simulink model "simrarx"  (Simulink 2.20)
settings: Solver=ode45  StartTime=0.0  StopTime=300  FixedStep=1  MaxStep=1  RelTol=1e-3  AbsTol=1e-6

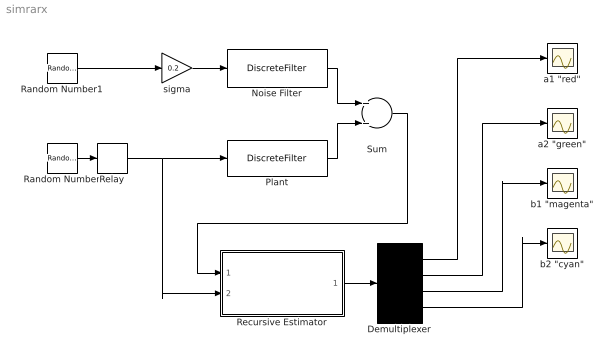
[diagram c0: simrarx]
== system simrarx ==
  Demultiplexer : Demux  Outputs=4
  Noise Filter : DiscreteFilter  Numerator=[1 -1 0.2]  Denominator=[1 -1.5 0.7]  SampleTime=1
  Plant : DiscreteFilter  Numerator=[1 0.5]  Denominator=[1 -1.5 0.7]  SampleTime=1
  Random Number : RandomNumber  Mean=0  Variance=1  Seed=123456789  SampleTime=1
  Random Number1 : RandomNumber  Mean=0  Variance=1  Seed=123459  SampleTime=1
  Recursive Estimator : Subsystem  mask(Recursive Estimator){nn=[2 2 1], ff=0.98, pdiag=10000, ts=1}
      mask prompts: nn "ARX model structure [na nb nk]  :"; ff "Forgetting factor  ff :"; pdiag "Íà÷àëíà ñòîéíîñò çà äèàãîíàëà íà êîâàðèàöèîííàòà ìàòðèöà  P  :"; ts "How often to sample points [sec] :"
      mask help: Recursive parameter estimation
      mask init:
      | nn=@1; ff=@2; pdiag=@3; ts=@4;
      | na=nn(1); d=na+nn(2); dm=sum(nn)-1;
      | i=[1:na  na+nn(3):dm];  ii=[1:dm];
  Relay : Relay  OnSwitchValue=eps  OffSwitchValue=eps  OnOutputValue=-1  OffOutputValue=1
  Sum : Sum  Inputs=++
  "a1 \"red\"" : Scope
  "a2 \"green\"" : Scope
  "b1 \"magenta\"" : Scope
  "b2 \"cyan\"" : Scope
  sigma : Gain  Gain=0.2
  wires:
  Random Number/1 -> Relay/1
  Random Number1/1 -> sigma/1
  sigma/1 -> Noise Filter/1
  Noise Filter/1 -> Sum/1
  Plant/1 -> Sum/2
  Sum/1 -> Recursive Estimator/1(y (k))
  Relay/1 -> Plant/1, Recursive Estimator/2(u (k))
  Recursive Estimator/1(tetha (k)) -> Demultiplexer/1
  Demultiplexer/1 -> "a1 \"red\""/1
  Demultiplexer/2 -> "a2 \"green\""/1
  Demultiplexer/3 -> "b1 \"magenta\""/1
  Demultiplexer/4 -> "b2 \"cyan\""/1

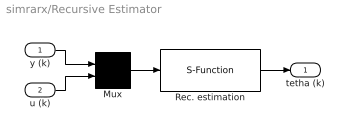
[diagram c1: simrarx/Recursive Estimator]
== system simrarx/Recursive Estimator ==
  y (k) : Inport  Port=1  PortWidth=-1  SampleTime=-1
  u (k) : Inport  Port=2  PortWidth=-1  SampleTime=-1
  Mux : Mux  Inputs=2
  Rec. estimation : S-Function  FunctionName=rarxm_sl  Parameters=na,ff,pdiag,ts,d,dm,i,ii  PortCounts=[]  SFunctionModules=''
  tetha (k) : Outport  Port=1
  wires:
  y (k)/1 -> Mux/1
  u (k)/1 -> Mux/2
  Mux/1 -> Rec. estimation/1
  Rec. estimation/1 -> tetha (k)/1
